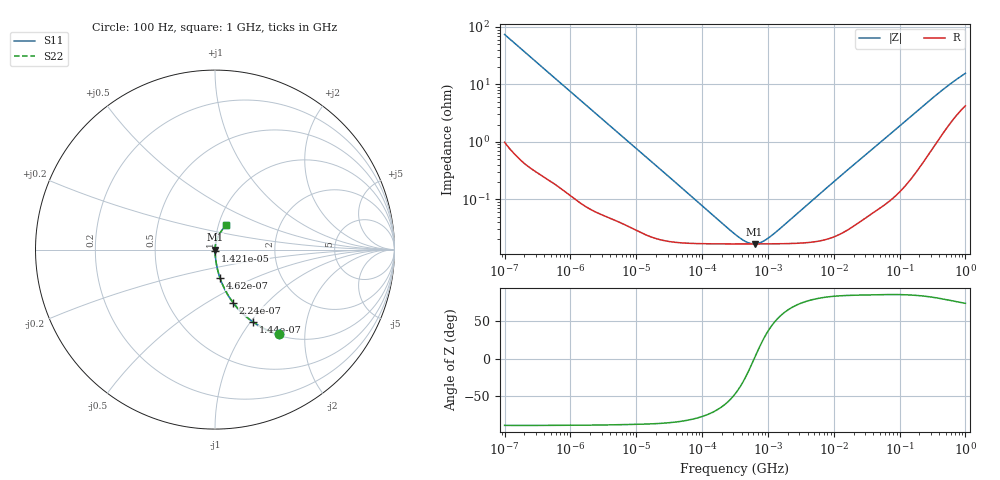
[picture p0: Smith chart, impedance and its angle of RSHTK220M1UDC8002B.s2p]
! RSHTK220M1UDC8002B  S-PARAMETER MODEL  (General Type)
! Model Generated by ELNA Corporation (http://www.ty-top.com)
! Version 1.0
! ELNA Control No.2403156
! Copyright (c) 2024 ELNA CO.,LTD. All Rights Reserved.
! Products Name : CONDUCTIVE POLYMER HYBRID ALUMINUM ELECTROLYTIC CAPACITORS
! Characteristics :
!  Capacitance  :  22uF  ,  Rated voltage  :  50V
!  Operating Temp. Range  :  -55 to +125 degC  ,  Endurance  :  6000hr at 125 degC
!  Dimension D  :  6.3mm  ,  Dimension L  :  5.8mm
! Frequency Range : 100Hz - 1GHz
! External Node Assignments :
!  1  o---| |---o  2
# MHz S RI R 50
!Freq[MHz].  S11 Real  S11 Imag  S21 Real  S21 Imag  S12 Real  S12 Imag  S22 Real  S22 Imag
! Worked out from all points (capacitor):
!   401 points, 100 Hz to 1 GHz, reference 50 ohm
!   read as one part in series: C = 21.5 uF near 108 Hz
!   lowest |Z| = 16.7 mohm at 627.3 kHz (marker M1)
!   series resonance near 618.4 kHz, so ESL is about 3.1 nH
!   S11 on the Smith chart (normalised r, x): 100 Hz: 1.02, -1.48; 144 Hz: 1.01, -1.03; 224 Hz: 1.01, -0.66; 462 Hz: 1.00, -0.32; 14.21 kHz: 1.00, -0.01; 1 GHz: 1.08, +0.30
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0.0001  0.3555 -0.4721  0.6445 0.4721  0.6445 0.4721  0.3555 -0.4721
0.000144  0.2123 -0.4032  0.7877 0.4032  0.7877 0.4032  0.2123 -0.4032
0.000224  0.1014 -0.2962  0.8986 0.2962  0.8986 0.2962  0.1014 -0.2962
0.000309  0.057 -0.2258  0.943 0.2258  0.943 0.2258  0.057 -0.2258
0.000462  0.0273 -0.1562  0.9727 0.1562  0.9727 0.1562  0.0273 -0.1562
0.000781  0.0105 -0.0946  0.9895 0.0946  0.9895 0.0946  0.0105 -0.0946
0.001488  0.00336 -0.0503  0.9966 0.0503  0.9966 0.0503  0.00336 -0.0503
0.003758  0.000886 -0.0201  0.9991 0.0201  0.9991 0.0201  0.000886 -0.0201
0.014207  0.000268 -0.00542  0.9997 0.00542  0.9997 0.00542  0.000268 -0.00542
0.022131  0.000212 -0.00349  0.9998 0.00349  0.9998 0.00349  0.000212 -0.00349
0.316228  0.000167 -0.000181  0.9998 0.000181  0.9998 0.000181  0.000167 -0.000181
0.473151  0.000167 -6.79e-05  0.9998 6.79e-05  0.9998 6.79e-05  0.000167 -6.79e-05
0.555904  0.000167 -2.67e-05  0.9998 2.67e-05  0.9998 2.67e-05  0.000167 -2.67e-05
0.627336  0.000167 3.63e-06  0.9998 -3.63e-06  0.9998 -3.63e-06  0.000167 3.63e-06
0.798914  0.000167 6.5e-05  0.9998 -6.5e-05  0.9998 -6.5e-05  0.000167 6.5e-05
1.102808  0.000168 0.000153  0.9998 -0.000153  0.9998 -0.000153  0.000168 0.000153
4.704354  0.000181 0.000936  0.9998 -0.000936  0.9998 -0.000936  0.000181 0.000936
69.9842  0.0011 0.0132  0.9989 -0.0132  0.9989 -0.0132  0.0011 0.0132
176.8072  0.00397 0.0326  0.996 -0.0326  0.996 -0.0326  0.00397 0.0326
395.8221  0.0158 0.0686  0.9842 -0.0686  0.9842 -0.0686  0.0158 0.0686
695.825  0.038 0.1069  0.962 -0.1069  0.962 -0.1069  0.038 0.1069
1000  0.0601 0.1353  0.9399 -0.1353  0.9399 -0.1353  0.0601 0.1353
